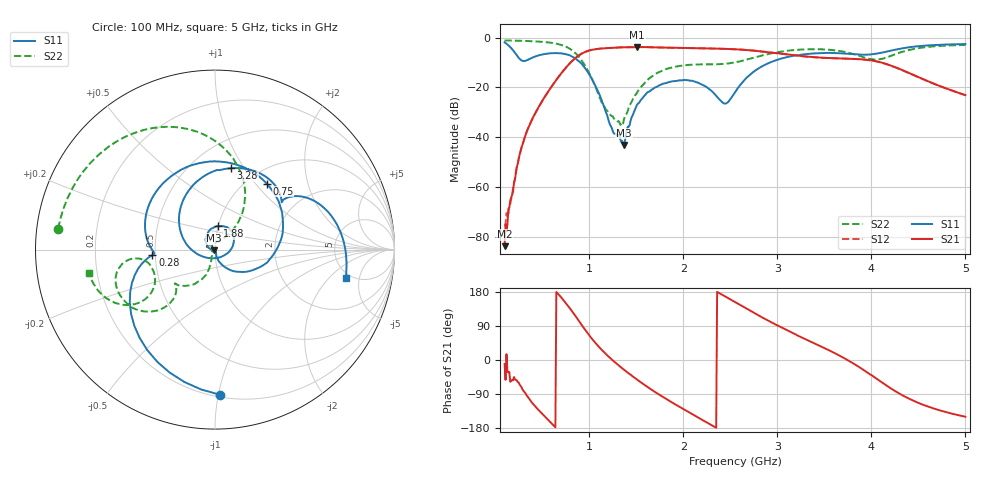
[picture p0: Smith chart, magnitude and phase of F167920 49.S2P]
!  2-Port S-parameters saved by WinCal
! VAR MeasName=S-Parameters (CALIBRATED_DATA) read from VNA (N5242A)
! VAR MeasDate=2016-11-22 9:57:56
! VAR NAME=F167920 49
! VAR FILENAME=F167920 49.S2P
! VAR DATE=2016-11-22 9:57:56
! VAR PHYS_PORTS=1,2
# Hz S DB R 50
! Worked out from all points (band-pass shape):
!   491 points, 100 MHz to 5 GHz, reference 50 ohm
!   highest |S21| = -3.74 dB at 1.51 GHz (marker M1); lowest = -83.8 dB at 100 MHz (marker M2)
!   |S21| within 3 dB of the highest: 904.2 MHz to 3.113 GHz (2.209 GHz wide, 110 % of centre)
!   lowest |S11| = -43.1 dB at 1.37 GHz (marker M3), VSWR 1.01, Z = 49.4 - j0.305 ohm
!   |S11| at or under -10 dB: 905.5 MHz to 2.919 GHz (2.014 GHz wide, 105 % of centre)
!   |S22| runs from -35.4 to -1.1 dB; largest |S21 - S12| = 0.0021
!   S11 on the Smith chart (normalised r, x): 100 MHz: 0.22, -1.01; 280 MHz: 0.48, -0.03; 750 MHz: 1.22, +1.15; 1.88 GHz: 1.00, +0.27; 3.28 GHz: 0.76, +0.88; 5 GHz: 4.52, -3.19
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1e8  -1.84 -88.1  -83.81 -10.6  -79.95 -26.7  -1.10 172.4
1.8e8  -4.61 -142.6  -63.16 -52.7  -63.25 -50.6  -1.15 166.3
2.8e8  -9.13 -175.0  -44.05 -72.0  -44.20 -72.4  -1.24 158.2
4.9e8  -6.82 138.2  -26.05 -139.5  -26.01 -139.5  -1.62 138.2
6.3e8  -6.17 93.4  -17.97 -175.0  -17.97 -175.0  -2.25 119.9
7.5e8  -6.61 51.8  -12.11 150.7  -12.11 150.7  -3.56 98.5
9.2e8  -10.48 -13.9  -6.35 92.6  -6.35 92.7  -9.18 61.0
1.17e9  -29.17 -77.9  -4.21 17.4  -4.21 17.4  -28.33 84.5
1.25e9  -37.55 -67.5  -4.04 -0.9  -4.04 -0.9  -31.57 124.5
1.37e9  -43.12 -153.7  -3.89 -25.7  -3.89 -25.8  -32.76 -137.4
1.51e9  -26.85 156.7  -3.74 -52.0  -3.75 -52.1  -22.00 -106.6
1.74e9  -19.21 107.7  -3.91 -90.9  -3.92 -90.9  -13.87 -117.7
1.88e9  -17.56 83.1  -4.05 -112.1  -4.05 -112.1  -11.95 -127.2
2.16e9  -18.14 31.4  -4.23 -152.2  -4.24 -152.2  -10.72 -138.7
2.44e9  -26.48 -78.5  -4.48 168.4  -4.47 168.4  -10.49 -136.3
2.55e9  -21.94 -151.9  -4.64 152.8  -4.65 152.8  -9.92 -132.7
2.84e9  -11.45 138.6  -5.54 112.2  -5.55 112.1  -7.11 -131.8
3.28e9  -6.69 78.8  -7.46 57.1  -7.49 57.1  -4.71 -151.2
3.37e9  -6.36 69.5  -7.76 46.6  -7.79 46.8  -4.62 -155.7
3.81e9  -6.63 37.7  -8.48 -9.3  -8.49 -9.1  -6.57 -173.7
4.19e9  -5.34 33.5  -10.96 -72.2  -10.98 -71.9  -7.55 -146.6
5e9  -2.56 -12.1  -23.07 -149.8  -23.06 -149.5  -2.94 -169.6
